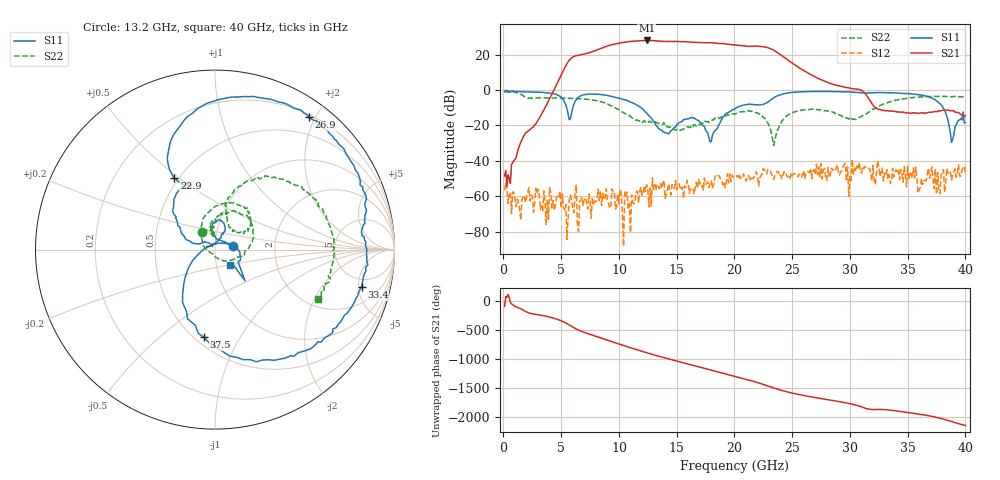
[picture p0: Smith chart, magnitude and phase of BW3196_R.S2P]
!Keysight Technologies,N5245A,MY52451660,A.10.49.11
!Date: Wednesday, January 24, 2018 09:20:35
!Correction: S11(Full 2 Port(1,2))
!S21(Full 2 Port(1,2))
!S12(Full 2 Port(1,2))
!S22(Full 2 Port(1,2))
!S2P File: Measurements: S11, S21, S12, S22:
# Hz S  dB  R 50
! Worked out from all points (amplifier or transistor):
!   400 points, 100 MHz to 40 GHz, reference 50 ohm
!   highest |S21| = 28.0 dB at 12.4 GHz (marker M1)
!   |S21| within 3 dB of that: 9.057 GHz to 20.67 GHz (11.61 GHz wide, 78.1 % of centre)
!   unconditionally stable (mu >= 1): start of sweep to end of sweep
!   at 6.7 GHz: K = 23.28, MAG = 24.4 dB, |S12| = -62.2 dB
!   at 20.1 GHz: K = 6.29, MAG = 26.2 dB, |S12| = -48.8 dB
!   at 40 GHz: K = 354.00, MAG = -12.4 dB, |S12| = -46.9 dB
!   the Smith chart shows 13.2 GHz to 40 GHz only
!   S11 on the Smith chart (normalised r, x): 13.2 GHz: 1.22, +0.05; 22.9 GHz: 0.48, +0.48; 26.9 GHz: 0.24, +1.92; 33.4 GHz: 3.79, -5.40; 37.5 GHz: 0.55, -0.72; 40 GHz: 1.16, -0.20
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1e8  -0.98 178.7  -48.50 -90.3  -56.66 -63.0  -0.12 -8.8
5.6e9  -13.60 -0.2  15.93 -38.9  -71.76 -97.4  -4.64 92.5
6.8e9  -2.97 142.5  20.04 -163.2  -60.81 -81.0  -4.99 53.8
8.6e9  -2.62 87.7  23.93 74.5  -58.26 124.4  -6.89 -13.7
9.9e9  -4.44 58.9  26.32 -12.7  -58.77 -11.9  -10.82 -68.6
1.12e10  -7.32 32.1  27.58 -96.4  -63.45 -44.9  -16.03 -136.0
1.24e10  -13.06 8.4  28.01 -169.5  -53.54 -106.0  -17.69 164.7
1.32e10  -19.96 11.8  27.78 143.6  -56.56 162.0  -18.19 125.5
1.34e10  -21.51 19.9  27.73 132.2  -54.34 -170.3  -18.70 117.1
1.45e10  -23.02 88.9  27.46 73.7  -59.26 154.7  -20.74 95.0
1.58e10  -16.58 90.2  27.20 4.1  -55.17 77.9  -21.23 102.2
1.78e10  -27.23 77.3  26.71 -99.1  -55.03 12.8  -18.34 94.2
1.9e10  -15.28 160.9  26.27 -163.7  -53.58 11.5  -15.15 86.7
2.01e10  -10.21 139.0  25.52 138.6  -48.75 -10.1  -13.35 71.8
2.15e10  -8.10 112.5  24.72 65.6  -49.79 -69.2  -12.02 36.5
2.29e10  -6.79 119.6  23.90 -23.0  -44.84 -145.6  -18.66 -28.5
2.44e10  -1.93 95.4  18.07 -116.6  -45.94 121.9  -15.51 115.3
2.67e10  -0.84 57.0  8.50 146.7  -50.16 56.7  -10.86 55.9
2.69e10  -0.87 54.5  7.74 139.9  -45.03 38.1  -10.96 54.0
3.34e10  -1.49 -14.3  -11.75 -79.6  -47.77 -27.3  -6.59 60.0
3.75e10  -6.15 -97.2  -12.23 155.3  -58.90 174.4  -3.59 2.3
4e10  -18.45 -46.8  -14.71 15.7  -46.92 -42.6  -3.93 -25.7
